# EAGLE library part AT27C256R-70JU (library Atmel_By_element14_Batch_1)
256K OTP EPROM
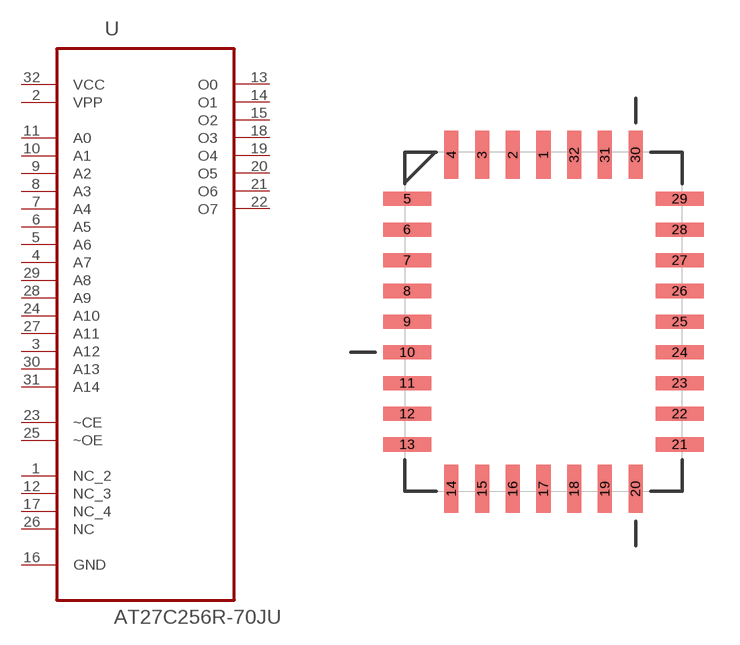
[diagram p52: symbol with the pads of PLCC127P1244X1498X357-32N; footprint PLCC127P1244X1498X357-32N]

Designator prefix U

## AT27C256R-70JU (DESCRIPTION: 256K OTP EPROM; MPN: AT27C256R-70JU; OC_FARNELL: 1095779; OC_NEWARK: 96K6554; PACKAGE: PLCC-32; SUPPLIER: Atmel Corporation)  [PLCC127P1244X1498X357-32N]
1  NC_2  nc
2  VPP  pwr
3  A12  in
4  A7  in
5  A6  in
6  A5  in
7  A4  in
8  A3  in
9  A2  in
10  A1  in
11  A0  in
12  NC_3  nc
13  O0  out
14  O1  out
15  O2  out
16  GND  pas
17  NC_4  nc
18  O3  out
19  O4  out
20  O5  out
21  O6  out
22  O7  out
23  ~CE  in
24  A10  in
25  ~OE  in
26  NC  nc
27  A11  in
28  A9  in
29  A8  in
30  A13  in
31  A14  in
32  VCC  pwr

## Footprint PLCC127P1244X1498X357-32N (pad centres in mm)
smd 0.584 x 1.981: 1 0,6.909; 2 -1.27,6.909; 3 -2.54,6.909; 4 -3.81,6.909; 14 -3.81,-6.909; 15 -2.54,-6.909; 16 -1.27,-6.909; 17 0,-6.909; 18 1.27,-6.909; 19 2.54,-6.909; 20 3.81,-6.909; 30 3.81,6.909; 31 2.54,6.909; 32 1.27,6.909
smd 1.981 x 0.584: 5 -5.639,5.08; 6 -5.639,3.81; 7 -5.639,2.54; 8 -5.639,1.27; 9 -5.639,0; 10 -5.639,-1.27; 11 -5.639,-2.54; 12 -5.639,-3.81; 13 -5.639,-5.08; 21 5.639,-5.08; 22 5.639,-3.81; 23 5.639,-2.54; 24 5.639,-1.27; 25 5.639,0; 26 5.639,1.27; 27 5.639,2.54; 28 5.639,3.81; 29 5.639,5.08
